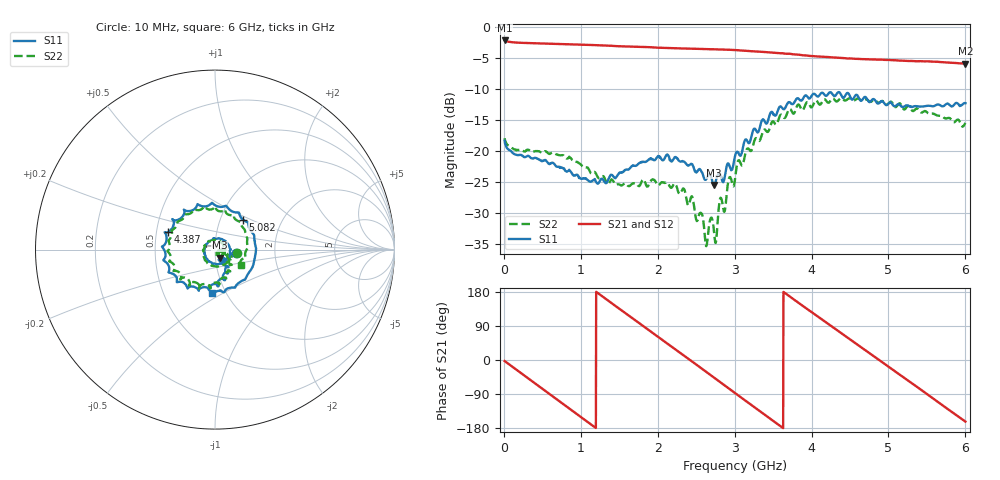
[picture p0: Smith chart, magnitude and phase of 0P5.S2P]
!Agilent Technologies,E5071C,MY46316741,A.11.02
!Date: Tue Oct 20 14:43:30 2020
!Data & Calibration Information:
!Freq	S11:SOLT4(ON)	S21:SOLT4(ON)	S12:SOLT4(ON)	S22:SOLT4(ON)
!PortZ  Port1:50+j0  Port2:50+j0
!Above PortZ is port z conversion or system Z0 setting when saving the data.
!When reading, reference impedance value at option line is always used.
# Hz S dB R 50
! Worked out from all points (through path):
!   1561 points, 10 MHz to 6 GHz, reference 50 ohm
!   highest |S21| = -2.22 dB at 10 MHz (marker M1); lowest = -6.0 dB at 6 GHz (marker M2)
!   group delay of S21, straight-line fit = 408 ps
!   lowest |S11| = -25.5 dB at 2.729 GHz (marker M3), VSWR 1.11, Z = 52.6 - j4.78 ohm
!   |S11| at or under -10 dB: start of sweep to end of sweep
!   |S22| runs from -35.4 to -11.5 dB; largest |S21 - S12| = 0.0056
!   S11 on the Smith chart (normalised r, x): 10 MHz: 1.27, -0.06; 4.387 GHz: 0.58, +0.12; 5.082 GHz: 1.28, +0.45; 6 GHz: 0.86, -0.44
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1e7  -18.40 -10.4  -2.22 -2.9  -2.27 -2.9  -17.99 -9.3
2.557436e8  -20.96 -40.2  -2.61 -39.3  -2.65 -39.3  -20.09 -32.6
5.360449e8  -21.51 -81.4  -2.71 -81.1  -2.75 -81.1  -20.08 -68.0
7.625897e8  -22.79 -119.6  -2.79 -114.8  -2.82 -114.9  -20.72 -100.8
1.012173e9  -24.53 -170.9  -2.89 -152.1  -2.92 -152.1  -22.39 -142.4
1.292474e9  -24.70 124.1  -3.01 166.2  -3.02 166.2  -24.17 158.4
1.588135e9  -23.05 54.7  -3.19 122.5  -3.21 122.4  -25.35 84.9
2.006667e9  -20.86 -13.1  -3.39 60.7  -3.40 60.6  -25.58 -4.0
2.367603e9  -22.12 -53.8  -3.53 7.7  -3.55 7.4  -27.34 -50.4
2.567269e9  -23.36 -63.9  -3.59 -21.7  -3.61 -22.1  -30.12 -60.3
2.628705e9  -24.60 -68.7  -3.60 -30.9  -3.64 -31.1  -35.39 -53.5
2.728538e9  -25.54 -59.1  -3.64 -45.7  -3.68 -45.9  -32.61 -11.3
3.005e9  -20.90 -52.9  -3.77 -87.0  -3.81 -87.2  -24.63 -23.5
3.243064e9  -16.62 -63.6  -3.96 -122.4  -3.99 -122.6  -19.02 -44.1
3.527205e9  -14.37 -89.5  -4.21 -164.5  -4.23 -164.6  -15.71 -70.9
4.007173e9  -11.04 -152.5  -4.73 125.5  -4.74 125.3  -12.94 -135.5
4.387308e9  -11.07 159.5  -5.04 70.7  -5.06 70.5  -11.55 -178.5
4.709846e9  -11.45 110.4  -5.24 24.6  -5.27 24.4  -11.72 143.3
5.001667e9  -12.40 59.8  -5.35 -17.8  -5.39 -17.8  -12.36 106.3
5.082301e9  -12.84 47.3  -5.41 -29.4  -5.45 -29.5  -12.92 98.5
5.523872e9  -12.75 -26.3  -5.59 -93.3  -5.61 -93.3  -14.02 43.0
6e9  -12.33 -93.6  -5.96 -162.5  -5.95 -162.4  -15.52 -31.1
